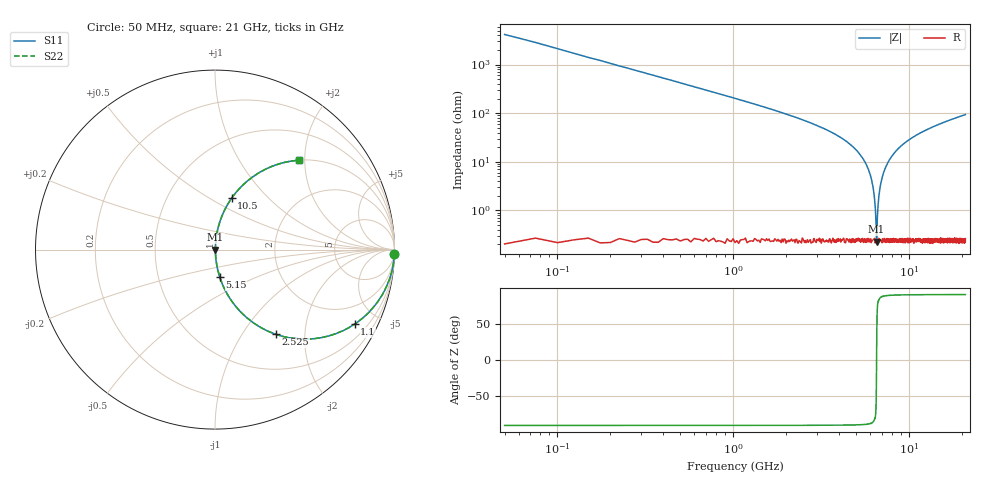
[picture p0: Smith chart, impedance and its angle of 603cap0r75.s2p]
! AVX Thin Film Operation		Date: November 2004
! Description: Accu-P® Series, Thin Film, SMD, RF Capacitor
! Part Number: 06035JR75ABT
! 50 MHz  -  10.05 GHz
! Serial Measurements
# MHZ S MA R 50
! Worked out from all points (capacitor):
!   839 points, 50 MHz to 21 GHz, reference 50 ohm
!   read as one part in series: C = 751 fF near 150 MHz
!   lowest |Z| = 228 mohm at 6.55 GHz (marker M1)
!   series resonance near 6.556 GHz, so ESL is about 780 pH
!   S11 on the Smith chart (normalised r, x): 50 MHz: -0, -85; 1.1 GHz: 1.00, -3.75; 2.525 GHz: 1.01, -1.43; 5.15 GHz: 1.00, -0.31; 10.5 GHz: 1.00, +0.63; 21 GHz: 1.01, +1.87
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50  1 -1.4  0.024 88.6  0.024 88.6  1 -1.4
225  0.994 -6.1  0.106 83.9  0.106 83.9  0.994 -6.1
400  0.982 -10.7  0.186 79.3  0.186 79.3  0.982 -10.7
1100  0.882 -28.1  0.47 61.9  0.47 61.9  0.882 -28.1
2525  0.581 -54.3  0.812 35.5  0.812 35.5  0.581 -54.3
3550  0.388 -66.8  0.919 22.9  0.919 22.9  0.388 -66.8
5150  0.155 -80.2  0.985 8.9  0.985 8.9  0.155 -80.2
5750  0.085 -83.5  0.994 4.9  0.994 4.9  0.085 -83.5
6125  0.044 -84.4  0.997 2.5  0.997 2.5  0.044 -84.4
6325  0.023 -82.8  0.997 1.3  0.997 1.3  0.023 -82.8
6475  0.008358 -72.9  0.998 0.5  0.998 0.5  0.008358 -72.9
6550  0.002466 -13.3  0.998 0.0  0.998 0.0  0.002466 -13.3
6625  0.007196 70.1  0.998 -0.4  0.998 -0.4  0.007196 70.1
6800  0.024 82.8  0.997 -1.4  0.997 -1.4  0.024 82.8
7050  0.047 84.4  0.997 -2.7  0.997 -2.7  0.047 84.4
7550  0.091 83.3  0.993 -5.2  0.993 -5.2  0.091 83.3
8250  0.148 80.6  0.987 -8.5  0.987 -8.5  0.148 80.6
10500  0.301 72.0  0.951 -17.5  0.951 -17.5  0.301 72.0
10525  0.302 72.0  0.951 -17.6  0.951 -17.6  0.302 72.0
14025  0.475 61.4  0.878 -28.4  0.878 -28.4  0.475 61.4
17525  0.596 53.2  0.801 -36.6  0.801 -36.6  0.596 53.2
21000  0.682 46.8  0.729 -43.0  0.729 -43.0  0.682 46.8
